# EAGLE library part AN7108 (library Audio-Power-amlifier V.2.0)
1-CHIP STEREO PRE-AMPLIFIER/POWER AMPLIFIER CIRCUIT 3V
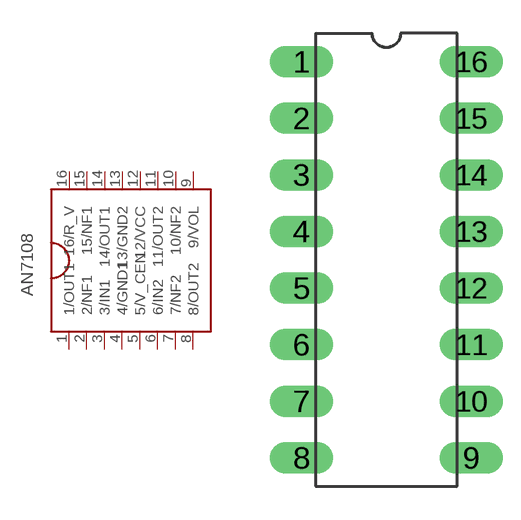
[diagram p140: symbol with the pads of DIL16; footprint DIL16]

Designator prefix IC

## AN7108  [DIL16]
1  1/OUT1  out
2  2/NF1  in
3  3/IN1  in
4  4/GND1  pwr
5  5/V_CEN  pwr
6  6/IN2  in
7  7/NF2  in
8  8/OUT2  out
9  9/VOL  in
10  10/NF2  in
11  11/OUT2  out
12  12/VCC  pwr
13  13/GND2  pwr
14  14/OUT1  out
15  15/NF1  in
16  16/R_V  in

## Footprint DIL16 (pad centres in mm)
drill 0.8 pad 1.422 long: 1 -3.81,8.89; 2 -3.81,6.35; 3 -3.81,3.81; 4 -3.81,1.27; 5 -3.81,-1.27; 6 -3.81,-3.81; 7 -3.81,-6.35; 8 -3.81,-8.89; 9 3.81,-8.89; 10 3.81,-6.35; 11 3.81,-3.81; 12 3.81,-1.27; 13 3.81,1.27; 14 3.81,3.81; 15 3.81,6.35; 16 3.81,8.89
